(* Logix 5000 AddOnInstructionDefinition export B256_NNRED; software revision 30.00 *)

ADD_ON_INSTRUCTION D_SHR   (* revision 1.0, vendor Ken Fischer, NSWCPD, C512 *)
// DINT bit shift right of the 32-bit argument Inp_A by Inp_B bits with paddding by zeros on the right
// Revision note:
// Rev1.0: TBD - Initial Release
VAR_IN_OUT
   Inp_A : DINT; {required}   // 64-bit Integer to be right circular rotated
END_VAR
VAR_INPUT
   Inp_B : INT; {required}   // Number of bits to shift
END_VAR
VAR_IN_OUT
   Out : DINT; {required}   // Result
END_VAR
VAR
   BSR_Cntrl : CONTROL := (LEN := 32);
   ONS : BOOL;
   Source_Bit : BOOL;
   Wrk_InpA : DINT[2];
END_VAR

ROUTINE Logic   (* ladder *)
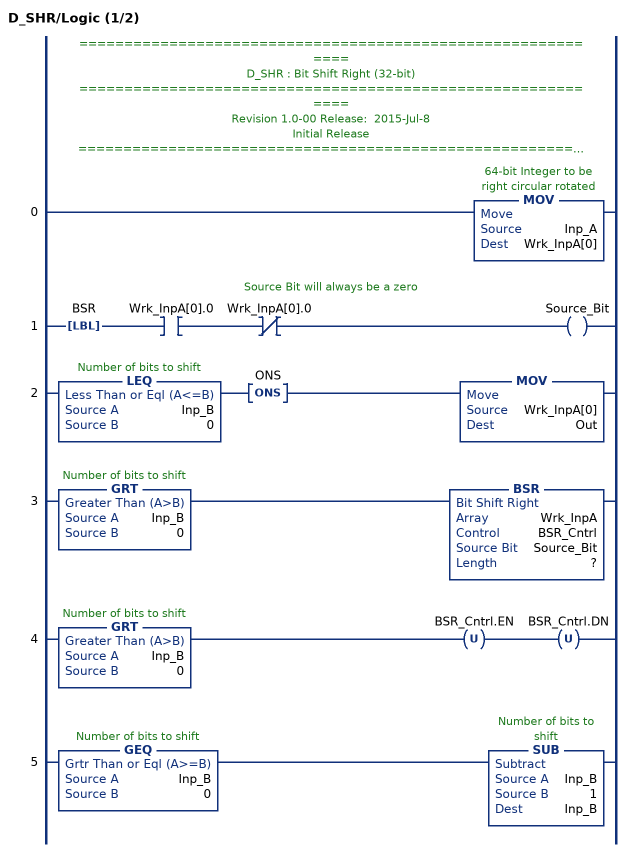
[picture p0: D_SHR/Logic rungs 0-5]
   // ============================================================
   // D_SHR : Bit Shift Right (32-bit)
   // ============================================================
   // Revision 1.0-00 Release:  2015-Jul-8
   // Initial Release
   // ============================================================
   // Performs a right bit shift of the 32-bit argument Inp_A by the
   // number of bits defined in the 16-bit argument Inp_B, with padding by zeros.
   0: MOV(Inp_A,Wrk_InpA[0]);
   // Source Bit will always be a zero
   1: LBL(BSR)XIC(Wrk_InpA[0].0)XIO(Wrk_InpA[0].0)OTE(Source_Bit);
   2: LEQ(Inp_B,0)ONS(ONS)MOV(Wrk_InpA[0],Out);
   3: GRT(Inp_B,0)BSR(Wrk_InpA,BSR_Cntrl,Source_Bit,?);
   4: GRT(Inp_B,0)OTU(BSR_Cntrl.EN)OTU(BSR_Cntrl.DN);
   5: GEQ(Inp_B,0)SUB(Inp_B,1,Inp_B);
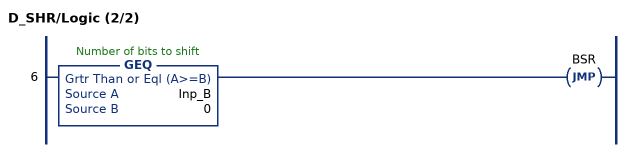
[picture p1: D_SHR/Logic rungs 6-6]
   6: GEQ(Inp_B,0)JMP(BSR);
END_ROUTINE
END_ADD_ON_INSTRUCTION

ADD_ON_INSTRUCTION B256_NNRED   (* revision 1.0 20170916, vendor Kenneth A. Fischer *)
// Reduce 256-bit integer stored in 43 pieces by propagating carries
// Revision note:
// Rev1.0: 20170916 - Initial Release
VAR_IN_OUT
   Inp_D : DINT[43]; {required}
END_VAR
VAR
   temp : DINT;
   i : INT;
   D_SHR : D_SHR;
END_VAR

ROUTINE Logic   (* ladder *)
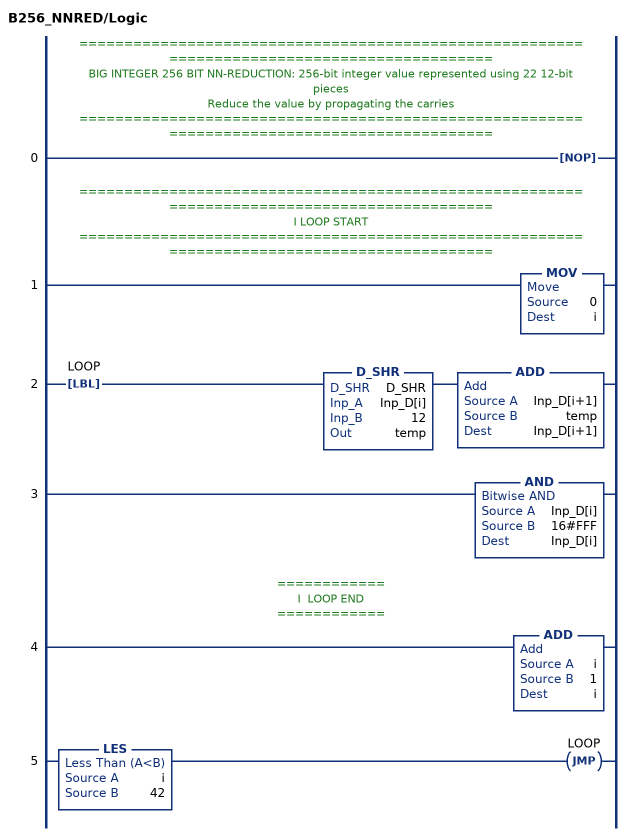
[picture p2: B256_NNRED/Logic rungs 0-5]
   // ============================================================================================
   // BIG INTEGER 256 BIT NN-REDUCTION: 256-bit integer value represented using 22 12-bit pieces
   // Reduce the value by propagating the carries
   // ============================================================================================
   0: NOP();
   // ============================================================================================
   // I LOOP START
   // ============================================================================================
   1: MOV(0,i);
   2: LBL(LOOP)D_SHR(D_SHR,Inp_D[i],12,temp)ADD(Inp_D[i+1],temp,Inp_D[i+1]);
   3: AND(Inp_D[i],16#FFF,Inp_D[i]);
   // ============
   // I  LOOP END
   // ============
   4: ADD(i,1,i);
   5: LES(i,42)JMP(LOOP);
END_ROUTINE
END_ADD_ON_INSTRUCTION
